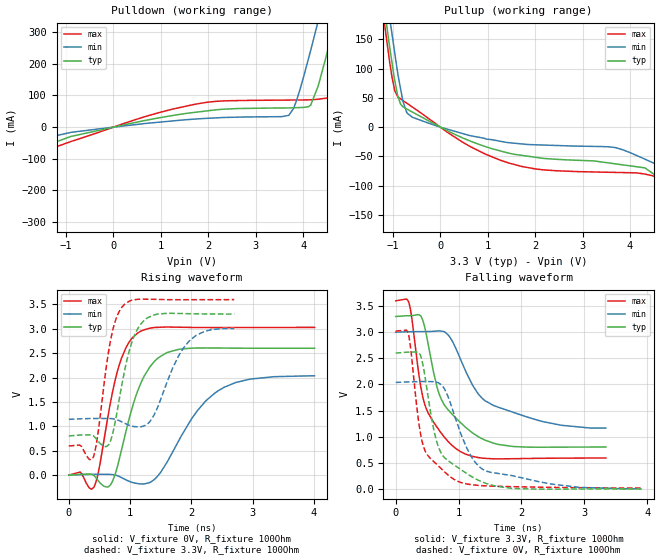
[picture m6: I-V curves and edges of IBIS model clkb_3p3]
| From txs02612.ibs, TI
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|   clkb_3p3 Model
[Model]   clkb_3p3
Model_type   Output
Polarity   Non-Inverting
Vmeas = 1.65
Vref = 1.65
Cref = 15pF
Rref = 100
|   typ   min   max
|   (nom PVT)   (fast PVT)   (slow PVT)
|C_comp from frequency sweep method (F=60MHz)
C_comp   5.696e-12   5.654e-12   5.833e-12
|ON state : BUFFER OUTPUT TURNED HIGH
|C_comp   5.696e-12   5.654e-12   5.833e-12
|OFF state: BUFFER OUTPUT TURNED LOW
|C_comp   4.940e-12   4.748e-12   7.128e-12
|C_comp from LC tank measurement(L=1nH)
|Resonant Frequency(Hz)   2.110e+09   2.130e+09   2.090e+09
|C_comp   5.695e-12   5.589e-12   5.805e-12
|ON state : BUFFER OUTPUT TURNED HIGH
|Resonant Frequency(Hz)   2.110e+09   2.130e+09   2.090e+09
|C_comp   5.695e-12   5.589e-12   5.805e-12
|OFF state: BUFFER OUTPUT TURNED LOW
|Resonant Frequency(Hz)   2.300e+09   2.300e+09   2.250e+09
|C_comp   4.793e-12   4.793e-12   5.008e-12
| Where nom  PVT is Nominal Process, 3.3V, 27C
|   Fast PVT is Strong Process,  3.6V, -40C
|   Slow PVT is Weak Process,   3V, 125C
[Voltage Range]   3.3   3   3.6
|Ambient Temperature   25   85   -40
|Junction Temperature
[Temperature Range]   27   125   -40
[Pullup Reference]   3.3   3   3.6
[Pulldown Reference]   0   0   0
[Power Clamp Reference]   3.3   3   3.6
[GND Clamp Reference]   0   0   0
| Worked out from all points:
|   slope of the pulldown table from 0 to 0.495 V, typ, clamps not added: 31.3 ohm
|   slope of the pullup table from 0 to 0.495 V, typ, clamps not added: 25.8 ohm
|   falling waveform, V_fixture 3.3V, R_fixture 100Ohm: 20-80 % time 492ps typ, 733ps min, 367ps max; typ from 3.3 V to 0.803 V
|   rising waveform, V_fixture 0V, R_fixture 100Ohm: 20-80 % time 395ps typ, 669ps min, 309ps max; typ from 0 V to 2.6 V
|   rising waveform, V_fixture 3.3V, R_fixture 100Ohm: 20-80 % time 262ps typ, 402ps min, 211ps max; typ from 0.803 V to 3.3 V
|   falling waveform, V_fixture 0V, R_fixture 100Ohm: 20-80 % time 384ps typ, 473ps min, 265ps max; typ from 2.6 V to 0 V
[Pulldown]
|   Voltage   I(typ)   I(min)   I(max)
-3.3V     -221mA     -127.8mA   -349.7mA
-2.98V    -143.6mA   -93.98mA   -241.8mA
-1.714V   -74.17mA   -43.71mA   -89.03mA
1.706V    46.56mA    25.33mA    71.86mA
3.693V    60.65mA    37.11mA    85.49mA
3.855V    61.5mA     81.75mA    85.69mA
4.158V    69.18mA    242.2mA    86.35mA
4.314V    128.9mA    333.5mA    88.07mA
4.507V    236.5mA    449.7mA    92.2mA
4.63V     312.9mA    526.2mA    126.2mA
4.889V    474.5mA    688.1mA    272.8mA
6.6V      1.576A     1.793A     1.365A
[Pullup]
|   Voltage   I(typ)   I(min)   I(max)
-3.3V     1.576A     1.596A     1.565A
-1.264V   254.2mA    302.7mA    229mA
-1.137V   178mA      225.3mA    152.7mA
-1.019V   110.1mA    159.3mA    85.47mA
-897.6mV  53.07mA    91.68mA    51.99mA
-792mV    35.11mA    45.38mA    45.66mA
-591mV    25.85mA    16.92mA    34.45mA
1.436V    -44.28mA   -26.53mA   -61.13mA
3.702V    -62.87mA   -35.15mA   -77.42mA
4.504V    -80.61mA   -61.72mA   -83.72mA
5.515V    -148.3mA   -101.1mA   -186.4mA
6.6V      -221mA     -143.7mA   -327.1mA
[Ramp]
R_load = 100
|   typ   min   max
dV/dt_r   1.5598/3.90909e-10   1.22319/6.66118e-10   1.79278/3.06509e-10
dV/dt_f   1.49804/4.92016e-10   1.11334/7.72633e-10   1.80144/3.63852e-10
[Falling Waveform]
V_fixture = 3.3V
V_fixture_min = 3V
V_fixture_max = 3.6V
R_fixture = 100Ohm
|   Time   V(typ)   V(min)   V(max)
0s        3.3V       3V         3.6V
212ps     3.314V     3.009V     3.558V
402ps     3.304V     3.011V     1.935V
498ps     2.89V      3.012V     1.504V
694ps     1.811V     3.024V     1.121V
952ps     1.365V     2.701V     779.3mV
1.242ns   1.057V     1.948V     619.4mV
1.554ns   877.9mV    1.6V       578.1mV
2.356ns   799.8mV    1.286V     588.2mV
3.344ns   803.2mV    1.165V     592.7mV
[Rising Waveform]
V_fixture = 0V
V_fixture_min = 0V
V_fixture_max = 0V
R_fixture = 100Ohm
|   Time   V(typ)   V(min)   V(max)
0s        81.38nV    4.99uV     13.03nV
184ps     20.73mV    10.58mV    65.15mV
410ps     -5.517mV   17.57mV    -242.3mV
680ps     -196.9mV   16.58mV    1.492V
860ps     519.7mV    -50.04mV   2.398V
1.168ns   1.866V     -177.7mV   2.946V
1.608ns   2.514V     277.9mV    3.035V
2.016ns   2.602V     1.179V     3.026V
2.448ns   2.604V     1.738V     3.023V
4.01ns    2.6V       2.036V     3.027V
[Rising Waveform]
V_fixture = 3.3V
V_fixture_min = 3V
V_fixture_max = 3.6V
R_fixture = 100Ohm
|   Time   V(typ)   V(min)   V(max)
0s        803.3mV    1.144V     598.5mV
400ps     807.1mV    1.161V     371.6mV
454ps     734.3mV    1.162V     669.7mV
672ps     675.6mV    1.161V     2.702V
790ps     1.315V     1.134V     3.267V
922ps     2.213V     1.057V     3.516V
1.062ns   2.837V     996.8mV    3.592V
1.292ns   3.229V     1.059V     3.604V
1.962ns   3.307V     2.745V     3.594V
2.7ns     3.3V       3.006V     3.596V
[Falling Waveform]
V_fixture = 0V
V_fixture_min = 0V
V_fixture_max = 0V
R_fixture = 100Ohm
|   Time   V(typ)   V(min)   V(max)
0s        2.6V       2.039V     3.021V
206ps     2.618V     2.049V     2.945V
368ps     2.604V     2.055V     1.26V
468ps     2.137V     2.057V     730.8mV
676ps     817.2mV    2.035V     445.8mV
776ps     601.1mV    1.917V     330.1mV
948ps     446.5mV    1.359V     169.9mV
1.194ns   246.8mV    639.9mV    84.71mV
1.442ns   105.9mV    343.1mV    60.2mV
3.91ns    10.74uV    4.537mV    18.09mV
